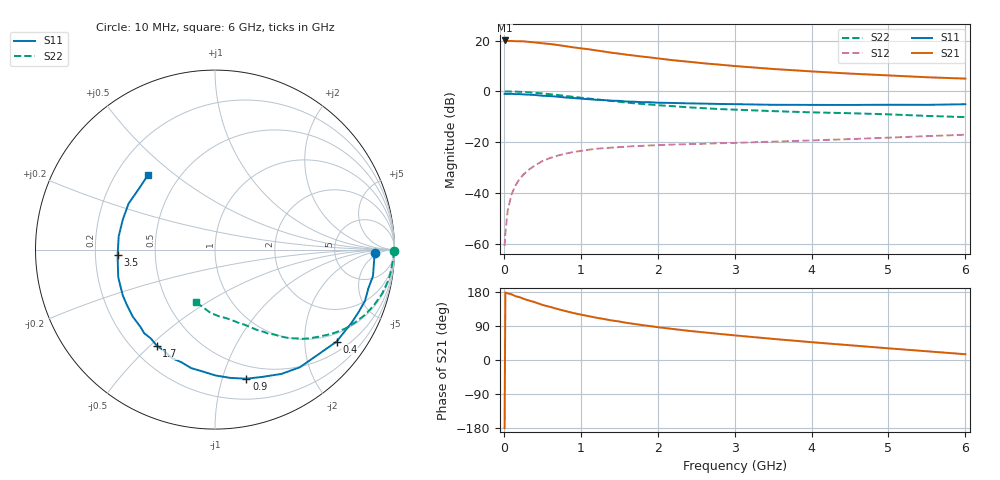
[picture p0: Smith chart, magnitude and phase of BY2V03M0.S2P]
! SIEMENS Small Signal Semiconductors
! BFY420
! Si NPN RF SIEGET Grounded Emitter Transistor in MICRO-X
! VCE = 2 V  IC = 3 mA
! Common Emitter S-Parameters:  October  1996
# GHz  S  MA  R  50
!  f  S11  S21  S12  S22
! GHz  MAG  ANG  MAG  ANG  MAG  ANG  MAG  ANG
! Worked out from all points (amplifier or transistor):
!   36 points, 10 MHz to 6 GHz, reference 50 ohm
!   highest |S21| = 20.0 dB at 10 MHz (marker M1)
!   |S21| within 3 dB of that: start of sweep to 977.2 MHz
!   unconditionally stable (mu >= 1): 3.599 GHz to end of sweep
!   at 250 MHz: K = 0.08, MSG = 26.3 dB, |S12| = -32.9 dB
!   at 1.4 GHz: K = 0.39, MSG = 18.7 dB, |S12| = -22.2 dB
!   at 6 GHz: K = 1.20, MAG = 8.4 dB, |S12| = -17.1 dB
!   S11 on the Smith chart (normalised r, x): 10 MHz: 17, -3; 400 MHz: 0.76, -2.80; 900 MHz: 0.38, -1.20; 1.7 GHz: 0.30, -0.52; 3.5 GHz: 0.30, -0.03; 6 GHz: 0.33, +0.40
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0.01  0.8906 -1.2  10.03 -179.8  0.0009 98.4  0.9952 -0.4
0.02  0.8893 -2.0  9.995 178.1  0.0016 86.7  0.9929 -1.0
0.05  0.8887 -4.9  9.79 175.8  0.0045 88.4  0.9949 -2.5
0.1  0.8923 -9.5  9.799 173.2  0.0094 85.0  0.9899 -5.0
0.15  0.8813 -14.2  9.704 168.6  0.014 81.0  0.9864 -7.5
0.2  0.8832 -18.9  9.671 166.0  0.0185 80.1  0.9815 -9.9
0.25  0.8721 -23.7  9.638 162.1  0.0227 76.0  0.9717 -12.3
0.4  0.8495 -37.1  9.187 152.7  0.0346 70.0  0.9386 -19.3
0.5  0.8191 -45.8  8.828 145.5  0.0424 65.1  0.9107 -23.6
0.6  0.8082 -54.2  8.551 140.1  0.0488 60.8  0.8789 -27.6
0.7  0.7853 -61.9  8.17 134.5  0.0544 56.7  0.8472 -31.4
0.9  0.7404 -76.3  7.355 124.1  0.0639 49.7  0.782 -37.5
1.1  0.7015 -89.7  6.746 115.7  0.0709 44.6  0.7236 -43.1
1.4  0.655 -106.6  5.749 104.5  0.078 38.3  0.6479 -49.7
1.7  0.6261 -121.2  5.041 95.1  0.0837 33.9  0.5809 -54.8
2  0.598 -134.1  4.453 86.6  0.0875 30.5  0.5338 -59.2
2.2  0.591 -140.9  4.096 81.8  0.0898 28.7  0.5111 -61.8
2.8  0.5646 -159.2  3.358 68.9  0.0955 25.5  0.4483 -68.7
3.5  0.5437 -176.6  2.756 55.7  0.1026 23.2  0.4085 -75.7
4.5  0.5402 161.9  2.236 38.9  0.115 20.5  0.3717 -86.8
5.5  0.543 141.1  1.894 23.0  0.1315 17.4  0.3288 -101.3
6  0.5582 132.1  1.781 15.2  0.1404 15.3  0.3114 -110.1
